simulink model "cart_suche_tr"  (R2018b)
settings: Solver=ode4  StartTime=0.0  StopTime=inf  FixedStep=1e-3  RelTol=1e-3
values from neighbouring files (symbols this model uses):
  sila = silaP_vc(i)    [suche_treni_vozik.m]    (also in mainSkript_mereniVozik.m = data_vozik.signals(1).values)
  smer = 1    [suche_treni_vozik.m]
undefined symbols (not defined in the file or in its folder): Humusoft, MF624
libraries: sldrtlib x7, simulink x4, powerlib_meascontrol x1

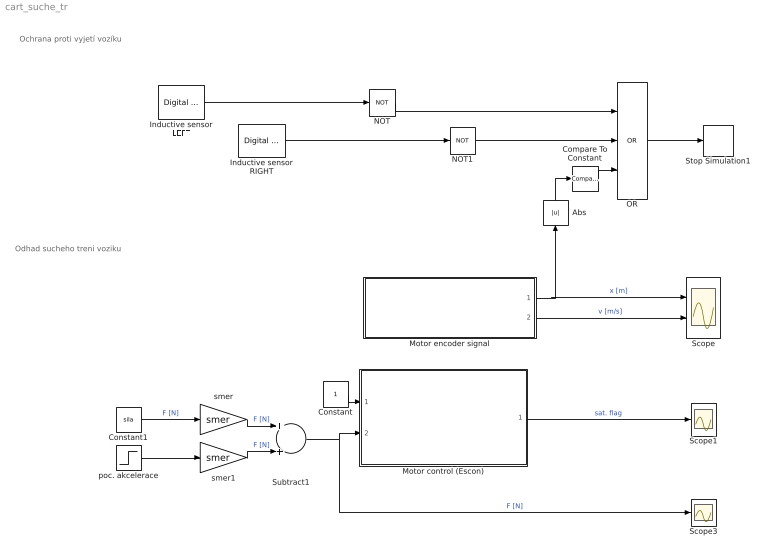
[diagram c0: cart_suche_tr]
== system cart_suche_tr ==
  note: Odhad sucheho treni voziku
  note: Ochrana proti vyjetí vozíku
  Abs : Abs
  Compare To Constant : simulink/Logic and Bit Operations/Compare To Constant  relop=>  const=0.75  OutDataTypeStr=boolean
  Constant : Constant
  Constant1 : Constant  Value=sila
  Inductive sensor LEFT : sldrtlib/Digital Input  SampleTime=0.001  MaxMissedTicks=1e6  ShowMissedTicks=off  YieldWhenWaiting=off  DrvName=Humusoft/MF624  DrvAddress=4294967295  DrvOptions=0  Channels=1  BitMode=1  DataType=1
  Inductive sensor RIGHT : sldrtlib/Digital Input  SampleTime=0.001  MaxMissedTicks=1e6  ShowMissedTicks=off  YieldWhenWaiting=off  DrvName=Humusoft/MF624  DrvAddress=4294967295  DrvOptions=0  Channels=2  BitMode=1  DataType=1
  Motor control (Escon) : Subsystem
  Motor encoder signal : Subsystem
  NOT : Logic  Operator=NOT  IconShape=distinctive  AllPortsSameDT=off  OutDataTypeStr=boolean
  NOT1 : Logic  Operator=NOT  IconShape=distinctive  AllPortsSameDT=off  OutDataTypeStr=boolean
  OR : Logic  Operator=OR  Inputs=3  IconShape=distinctive  AllPortsSameDT=off  OutDataTypeStr=boolean
  Scope : Scope  NumInputPorts=2
  Scope1 : Scope
  Scope3 : Scope
  Stop Simulation1 : Stop
  Subtract1 : Sum
  poc. akcelerace : Step  Time=0.05  Before=8  After=0  SampleTime=0
  smer : Gain  Gain=smer
  smer1 : Gain  Gain=smer
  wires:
  Constant/1 -> Motor control (Escon)/1(ENABLE)
  Motor control (Escon)/1(saturation flag) -> Scope1/1  "sat. flag"
  Motor encoder signal/1(x [m]) -> Abs/1, Scope/1  "x [m]"
  Motor encoder signal/2(v [m/s]) -> Scope/2  "v [m/s]"
  NOT1/1 -> OR/2
  NOT/1 -> OR/1
  Inductive sensor LEFT/1 -> NOT/1
  Inductive sensor RIGHT/1 -> NOT1/1
  OR/1 -> Stop Simulation1/1
  Constant1/1 -> smer/1  "F [N]"
  Subtract1/1 -> Scope3/1, Motor control (Escon)/2(Ref strength [N])  "F [N]"
  smer/1 -> Subtract1/1  "F [N]"
  poc. akcelerace/1 -> smer1/1
  smer1/1 -> Subtract1/2  "F [N]"
  Compare To Constant/1 -> OR/3
  Abs/1 -> Compare To Constant/1

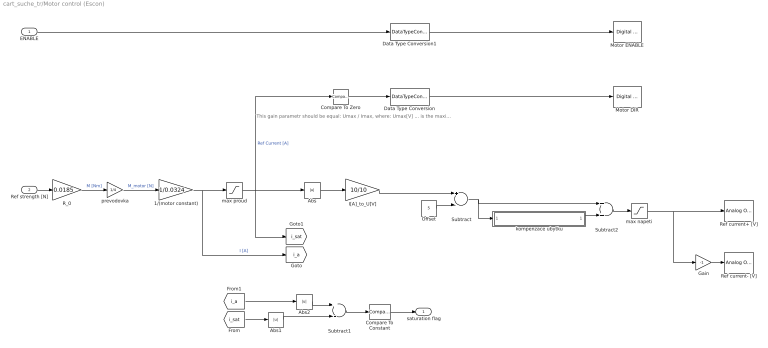
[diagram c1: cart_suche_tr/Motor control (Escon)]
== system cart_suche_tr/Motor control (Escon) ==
  note: This gain parametr should be equal: Umax / Imax, where: Umax[V] ... is the maximum absolute value of the output voltage (for MF624 Umax = 10 V ... think about MF624 isolation board voltage reduction ) Imax[A] ... is the maximum allowed current
  ENABLE : Inport
  Ref strength [N] : Inport  Port=2
  1/(motor constant) : Gain  Gain=1/0.0324
  Abs : Abs
  Abs1 : Abs
  Abs2 : Abs
  Compare To Constant : simulink/Logic and Bit Operations/Compare To Constant  relop=>  const=1e-8  OutDataTypeStr=boolean
  Compare To Zero : simulink/Logic and Bit Operations/Compare To Zero  relop=>=  OutDataTypeStr=boolean
  Data Type Conversion : DataTypeConversion  OutDataTypeStr=boolean
  Data Type Conversion1 : DataTypeConversion  OutDataTypeStr=boolean
  Gain : Gain  Gain=-1
  I[A]_to_U[V] : Gain  Gain=10/10
  Motor DIR : sldrtlib/Digital Output  SampleTime=0.001  MaxMissedTicks=1e6  ShowMissedTicks=off  YieldWhenWaiting=off  DrvName=Humusoft/MF624  DrvAddress=4294967295  DrvOptions=0  Channels=5  BitMode=1  InitialValue=[]  FinalValue=[]
  Motor ENABLE : sldrtlib/Digital Output  SampleTime=0.001  MaxMissedTicks=1e6  ShowMissedTicks=off  YieldWhenWaiting=off  DrvName=Humusoft/MF624  DrvAddress=4294967295  DrvOptions=0  Channels=2  BitMode=1  InitialValue=0  FinalValue=0
  Offset : Constant  Value=5
  R_0 : Gain  Gain=0.0185
  Ref current+ [V] : sldrtlib/Analog Output  SampleTime=0.001  MaxMissedTicks=1e6  ShowMissedTicks=off  YieldWhenWaiting=off  DrvName=Humusoft/MF624  DrvAddress=4294967295  DrvOptions=0  Channels=6  RangeMode=1  VoltRange=1  InitialValue=-5  FinalValue=-5
  Ref current- [V] : sldrtlib/Analog Output  SampleTime=0.001  MaxMissedTicks=1e6  ShowMissedTicks=off  YieldWhenWaiting=off  DrvName=Humusoft/MF624  DrvAddress=4294967295  DrvOptions=0  Channels=5  RangeMode=1  VoltRange=1  InitialValue=5  FinalValue=5
  Subtract : Sum  Inputs=+-
  Subtract1 : Sum  Inputs=+-
  Subtract2 : Sum
  kompenzace ubytku : Subsystem
  max napeti : Saturate  UpperLimit=5.5  LowerLimit=-5.5
  max proud : Saturate  UpperLimit=10  LowerLimit=-10
  prevodovka : Gain  Gain=1/4
  saturation flag : Outport
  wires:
  Data Type Conversion/1 -> Motor DIR/1
  Abs/1 -> I[A]_to_U[V]/1
  Gain/1 -> Ref current- [V]/1
  Compare To Zero/1 -> Data Type Conversion/1
  Data Type Conversion1/1 -> Motor ENABLE/1
  I[A]_to_U[V]/1 -> Subtract/1
  1/(motor constant)/1 -> max proud/1, [i_a]  "I [A]"
  max proud/1 -> Abs/1, Compare To Zero/1, [i_sat]  "Ref Current [A]"
  Ref strength [N]/1 -> R_0/1
  max napeti/1 -> Gain/1, Ref current+ [V]/1
  Offset/1 -> Subtract/2
  ENABLE/1 -> Data Type Conversion1/1
  Subtract2/1 -> max napeti/1
  kompenzace ubytku/1(error compensation [V]) -> Subtract2/2
  Subtract/1 -> kompenzace ubytku/1(voltage out [V]), Subtract2/1
  R_0/1 -> prevodovka/1  "M [Nm]"
  Abs1/1 -> Subtract1/2
  Abs2/1 -> Subtract1/1
  Subtract1/1 -> Compare To Constant/1
  Compare To Constant/1 -> saturation flag/1
  [i_a] -> Abs2/1
  [i_sat] -> Abs1/1
  prevodovka/1 -> 1/(motor constant)/1  "M_motor [N]"

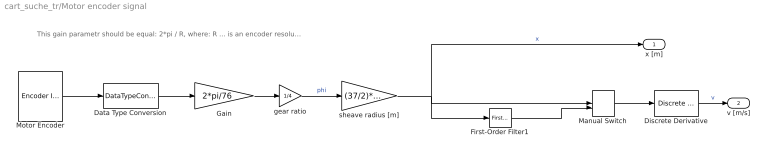
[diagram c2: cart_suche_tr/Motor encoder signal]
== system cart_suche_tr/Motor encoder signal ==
  note: This gain parametr should be equal: 2*pi / R, where: R ... is an encoder resolution
  Data Type Conversion : DataTypeConversion  OutDataTypeStr=double
  Discrete Derivative : simulink/Discrete/Discrete Derivative  gainval=1.0  ICPrevScaledInput=0.0  OutMin=[]  OutMax=[]  OutDataType=fixdt(1, 16)  OutScaling=2^-10  DoSatur=off
  First-Order Filter1 : powerlib_meascontrol/Filters/First-Order Filter  FilterType=Lowpass  Tc=0.004  Ts=0.001  Initialize=on  Vac_Init=[0, 0, 60]  Vdc_Init=0  PlotResponse=off  FreqRange="[0,  200,  1]"
  Gain : Gain  Gain=2*pi/76
  Manual Switch : ManualSwitch  CurrentSetting=0
  Motor Encoder : sldrtlib/Encoder Input  SampleTime=0.001  MaxMissedTicks=1e8  ShowMissedTicks=off  YieldWhenWaiting=off  DrvName=Humusoft/MF624  DrvAddress=4294967295  DrvOptions=0  Channels=3  QuadMode=3  IndexPulse=2  InputFilter=Inf  DataType=7
  gear ratio : Gain  Gain=1/4
  sheave radius [m] : Gain  Gain=(37/2)*1e-3
  x [m] : Outport
  v [m/s] : Outport  Port=2
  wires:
  Motor Encoder/1 -> Data Type Conversion/1
  Discrete Derivative/1 -> v [m/s]/1  "v"
  Data Type Conversion/1 -> Gain/1
  Gain/1 -> gear ratio/1
  sheave radius [m]/1 -> First-Order Filter1/1, Manual Switch/1, x [m]/1  "x"
  gear ratio/1 -> sheave radius [m]/1  "phi"
  First-Order Filter1/1 -> Manual Switch/2
  Manual Switch/1 -> Discrete Derivative/1

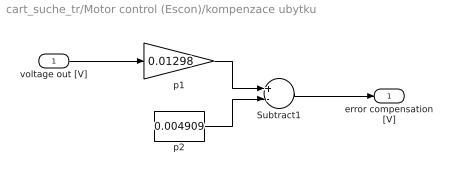
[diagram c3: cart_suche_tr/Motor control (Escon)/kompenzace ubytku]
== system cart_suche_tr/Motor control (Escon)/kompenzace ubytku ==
  voltage out [V] : Inport
  Subtract1 : Sum  Inputs=+-
  p1 : Gain  Gain=0.01298
  p2 : Constant  Value=0.004909
  error compensation [V] : Outport
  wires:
  p1/1 -> Subtract1/1
  p2/1 -> Subtract1/2
  Subtract1/1 -> error compensation [V]/1
  voltage out [V]/1 -> p1/1
